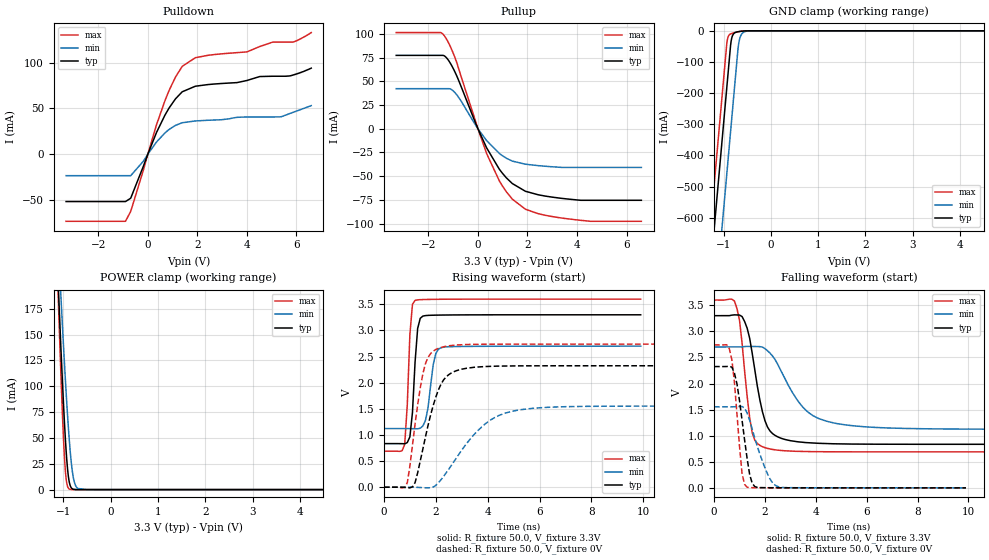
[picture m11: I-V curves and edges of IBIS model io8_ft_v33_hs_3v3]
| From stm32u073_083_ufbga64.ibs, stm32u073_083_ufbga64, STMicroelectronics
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[Model]   io8_ft_v33_hs_3v3
Model_type I/O
Polarity   Non-Inverting
Enable   Active-Low
| CAP_THRESHOLD on pad IOFT is "UDTCAPC" :
| Rising=30.0% of vddiom   Falling=70.0% of vddiom
| C_comp min and max val. don't necessarily correlate with the min and max pvt
| but are the smallest and greatest pad capacitance found.
| var   typ   min   max
C_comp   2.27946pF  2.25176pF  2.68147pF
|C_comp_pullup   1.26022pF  1.27543pF  1.50397pF
|C_comp_pulldown   1.01924pF  976.32715fF  1.17750pF
Vinl = 810.0mV
Vinh = 2.52V
Vmeas = 1.65V   | Reference voltage for timing measurements
Cref  = 50.0pF   | Timing specification test load capacitance value
Rref  = 100.0MOhm   | Timing specification test load resistance value
Vref  = 1.65V   | Timing specification test load voltage
[Model Spec]
| TIME_THRESHOLD on pin ZIV33M is "CMOS" :
| Rising=50.0% of vddiom   Falling=50.0% of vddiom
Vinl 1.34770V 1.11470V 1.44970V
Vinh 1.77530V 1.49030V 1.90330V
| variable   typ   min   max
[Temperature Range] 25.0 140.0 -40.0
| variable   typ   min   max
[Voltage Range] 3.3V 2.7V 3.6V
| variable   typ   min   max
[POWER Clamp Reference] 3.3V 2.7V 3.6V
| variable   typ   min   max
[GND Clamp Reference] 0V 0V 0V
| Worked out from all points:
|   slope of the pulldown table from 0 to 0.495 V, typ, clamps not added: 15.6 ohm
|   slope of the pullup table from 0 to 0.495 V, typ, clamps not added: 18.7 ohm
|   GND clamp passes 1 mA (typ) near -0.60 V on its own axis
|   POWER clamp passes 1 mA (typ) near -0.81 V on its own axis
|   rising waveform, R_fixture 50.0, V_fixture 3.3V: 20-80 % time 186ps typ, 252ps min, 157ps max; typ from 0.835 V to 3.3 V
|   falling waveform, R_fixture 50.0, V_fixture 3.3V: 20-80 % time 557ps typ, 1.25ns min, 380ps max; typ from 3.3 V to 0.835 V
|   rising waveform, R_fixture 50.0, V_fixture 0V: 20-80 % time 713ps typ, 1.54ns min, 476ps max; typ from 0 V to 2.33 V
|   falling waveform, R_fixture 50.0, V_fixture 0V: 20-80 % time 389ps typ, 635ps min, 286ps max; typ from 2.33 V to 0 V
[POWER Clamp]
-3.3V     2.991A     2.546A     3.694A
-1.11V    202.2mA    242.3mA    190.9mA
-1.09V    180mA      223.6mA    163.4mA
-1.05V    136.9mA    187mA      110.9mA
-1.01V    96.55mA    151.6mA    64.02mA
-970mV    60.39mA    117.9mA    27.41mA
-930mV    31.08mA    86.54mA    7.282mA
-860mV    4.779mA    40.5mA     315.2uA
-810mV    823.2uA    18.15mA    29.21uA
-750mV    88.98uA    4.952mA    1.667uA
-510mV    11.25nA    8.405uA    48.77pA
6.6V      0A         0A         0A
[GND Clamp]
-3.3V     -4.209A    -4.487A    -4.067A
-1.41V    -996.3mA   -1.274A    -854.3mA
-1.25V    -724.3mA   -1.002A    -582.3mA
-1.21V    -656.3mA   -933.6mA   -514.3mA
-930mV    -180.3mA   -457.6mA   -39.53mA
-900mV    -129.3mA   -406.6mA   -18.05mA
-840mV    -33.79mA   -304.6mA   -9.105mA
-790mV    -10.15mA   -219.6mA   -6.665mA
-680mV    -2.476mA   -41.57mA   -2.768mA
-630mV    -1.406mA   -13.77mA   -1.51mA
-530mV    -268.4uA   -1.762mA   -214.9uA
6.6V      830.6pA    196nA      594.5pA
| variable   typ   min   max
[Pullup Reference] 3.3V 2.7V 3.6V
| variable   typ   min   max
[Pulldown Reference] 0V 0V 0V
[Pullup]
-3.3V     77.35mA    42.24mA    101.4mA
-1.51V    77.35mA    42.24mA    101.4mA
-1.34V    76.54mA    42.24mA    97.42mA
-1.1V     68.45mA    41.76mA    85.85mA
-870mV    56.55mA    36.27mA    70.84mA
350mV     -20.12mA   -12.47mA   -26.09mA
860mV     -42.5mA    -25.9mA    -54.7mA
1.39V     -57.81mA   -34.14mA   -74.25mA
1.92V     -65.96mA   -37.41mA   -84.89mA
2.96V     -71.97mA   -40.03mA   -92.43mA
4.54V     -75.45mA   -40.79mA   -97.6mA
6.6V      -75.45mA   -40.79mA   -97.6mA
[Pulldown]
-3.3V     -51.64mA   -23.39mA   -73.18mA
-900mV    -51.64mA   -23.39mA   -73.04mA
-690mV    -47.97mA   -23.39mA   -62.4mA
350mV     23.63mA    13.27mA    31.99mA
690mV     42.49mA    23.17mA    58.21mA
1.12V     60.48mA    31.51mA    84.25mA
1.39V     68.1mA     34.34mA    95.86mA
1.92V     74.17mA    36.28mA    105.3mA
4V        80.41mA    40.64mA    111.6mA
5.39V     85.07mA    40.9mA     122.4mA
5.88V     86.5mA     45.8mA     122.4mA
6.6V      93.9mA     53mA       132.7mA
[Ramp]
dV/dt_r 1.39485V/712.42016ps 931.93282mV/1.53552ns 1.64323V/473.86145ps
dV/dt_f 1.47909V/551.1532ps 946.45174mV/1.2459ns 1.74612V/369.08999ps
R_load = 50.0
| Removed startup time: 0s 0s 0s  .
| Removed end time: 9.9ns.
[Rising Waveform]
R_fixture   = 50.0
V_fixture   = 3.3V
V_fixture_min = 2.7V
V_fixture_max = 3.6V
0s        834.8mV    1.123V     689.8mV
800ps     831.6mV    1.123V     816.8mV
900ps     854.4mV    1.122V     1.577V
1ns       963.8mV    1.122V     2.923V
1.2ns     2.394V     1.12V      3.576V
1.4ns     3.233V     1.13V      3.59V
1.6ns     3.285V     1.276V     3.593V
2ns       3.293V     2.559V     3.596V
2.2ns     3.295V     2.669V     3.597V
9.9ns     3.3V       2.7V       3.6V
| Removed startup time: 0s 0s 0s  .
| Removed end time: 19.9ns.
[Falling Waveform]
R_fixture   = 50.0
V_fixture   = 3.3V
V_fixture_min = 2.7V
V_fixture_max = 3.6V
0s        3.3V       2.7V       3.6V
800ps     3.316V     2.7V       3.58V
1ns       3.312V     2.7V       3.209V
1.3ns     3.061V     2.711V     1.753V
1.5ns     2.577V     2.71V      1.052V
2ns       1.288V     2.668V     770.1mV
2.4ns     1.005V     2.457V     728.9mV
3.5ns     872.4mV    1.541V     697mV
4.8ns     843.8mV    1.235V     691.1mV
19.9ns    834.9mV    1.123V     689.8mV
| Removed startup time: 0s 0s 0s  .
| Removed end time: 19.9ns.
[Rising Waveform]
R_fixture   = 50.0
V_fixture   = 0V
V_fixture_min = 0V
V_fixture_max = 0V
0s        -9.489uV   -14.68uV   3.008uV
900ps     -11.06mV   72.31uV    85.24mV
1.2ns     88.28mV    -18.83uV   1.209V
1.4ns     498.4mV    -5.61mV    1.901V
1.6ns     961.4mV    -11.21mV   2.365V
2ns       1.726V     35.81mV    2.635V
2.3ns     2.054V     206.6mV    2.688V
3.8ns     2.308V     1.168V     2.737V
5.3ns     2.323V     1.485V     2.738V
19.9ns    2.325V     1.553V     2.739V
| Removed startup time: 0s 0s 0s  .
| Removed end time: 9.9ns.
[Falling Waveform]
R_fixture   = 50.0
V_fixture   = 0V
V_fixture_min = 0V
V_fixture_max = 0V
0s        2.325V     1.553V     2.739V
600ps     2.33V      1.553V     2.665V
800ps     2.199V     1.554V     2.022V
1.1ns     1.297V     1.56V      275.3mV
1.3ns     558.9mV    1.434V     11.77mV
1.4ns     252mV      1.292V     5.72mV
1.6ns     24.82mV    952.9mV    3.364mV
2.1ns     2.997mV    269.2mV    1.766mV
2.5ns     1.931mV    25.84mV    1.163mV
9.9ns     15.12uV    54.11uV    6.017uV
